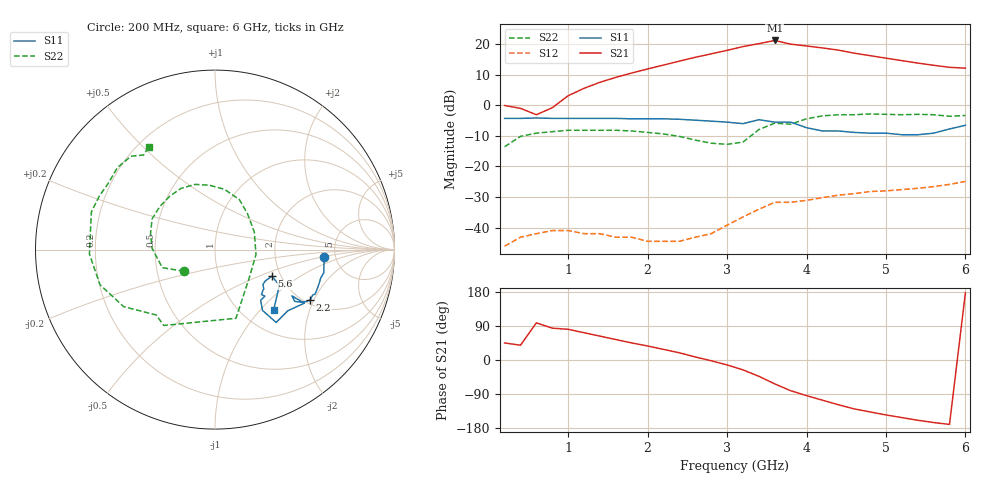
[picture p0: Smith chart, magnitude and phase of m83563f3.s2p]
!	MGA-83563 S PARAMETERS
!	Vd = 3 V L=0.0 nH  LAST UPDATED 10-15-97
# ghz	s ma r	50
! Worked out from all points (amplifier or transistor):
!   30 points, 200 MHz to 6 GHz, reference 50 ohm
!   highest |S21| = 21.2 dB at 3.6 GHz (marker M1)
!   |S21| within 3 dB of that: 3.038 GHz to 4.358 GHz (1.321 GHz wide, 35.7 % of centre)
!   unconditionally stable (mu >= 1): start of sweep to end of sweep
!   at 1.2 GHz: K = 17.39, MAG = 8.3 dB, |S12| = -41.9 dB
!   at 3.2 GHz: K = 2.77, MAG = 20.5 dB, |S12| = -36.5 dB
!   at 6 GHz: K = 1.33, MAG = 15.0 dB, |S12| = -24.9 dB
!   S11 on the Smith chart (normalised r, x): 200 MHz: 4.05, -0.55; 2.2 GHz: 2.13, -1.87; 5.6 GHz: 1.80, -0.61; 6 GHz: 1.37, -1.19
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0.2  0.61 -4.0  0.99 45.0  0.005 62.0  0.21 -145.0
0.4  0.61 -5.0  0.89 39.0  0.007 48.0  0.31 -161.0
0.6  0.62 -12.0  0.7 98.0  0.008 35.0  0.35 179.0
1.2  0.61 -21.0  1.89 72.0  0.008 28.0  0.39 142.0
1.8  0.6 -25.0  3.36 45.0  0.007 37.0  0.38 107.0
2.2  0.6 -28.0  4.53 28.0  0.006 57.0  0.34 81.0
2.4  0.59 -29.0  5.25 19.0  0.006 69.0  0.31 64.0
2.8  0.55 -32.0  6.9 -2.0  0.008 97.0  0.24 24.0
3  0.53 -33.0  7.87 -13.0  0.011 109.0  0.23 -7.0
3.2  0.5 -31.0  9.07 -26.0  0.015 112.0  0.25 -41.0
3.4  0.58 -31.0  10.13 -43.0  0.02 107.0  0.4 -73.0
3.6  0.53 -40.0  11.42 -63.0  0.026 101.0  0.51 -124.0
3.8  0.53 -50.0  9.95 -81.0  0.026 94.0  0.49 -132.0
4  0.43 -52.0  9.28 -94.0  0.028 93.0  0.6 -148.0
4.2  0.38 -48.0  8.62 -106.0  0.031 91.0  0.67 -163.0
4.4  0.38 -43.0  7.95 -118.0  0.034 87.0  0.7 -178.0
4.6  0.36 -44.0  7.08 -129.0  0.036 84.0  0.7 173.0
5  0.35 -39.0  5.87 -145.0  0.04 78.0  0.71 155.0
5.2  0.33 -36.0  5.35 -152.0  0.042 76.0  0.7 148.0
5.6  0.35 -25.0  4.49 -165.0  0.047 75.0  0.7 132.0
5.8  0.41 -29.0  4.16 -170.0  0.051 73.0  0.66 127.0
6  0.47 -46.0  4.03 177.0  0.057 64.0  0.68 123.0
